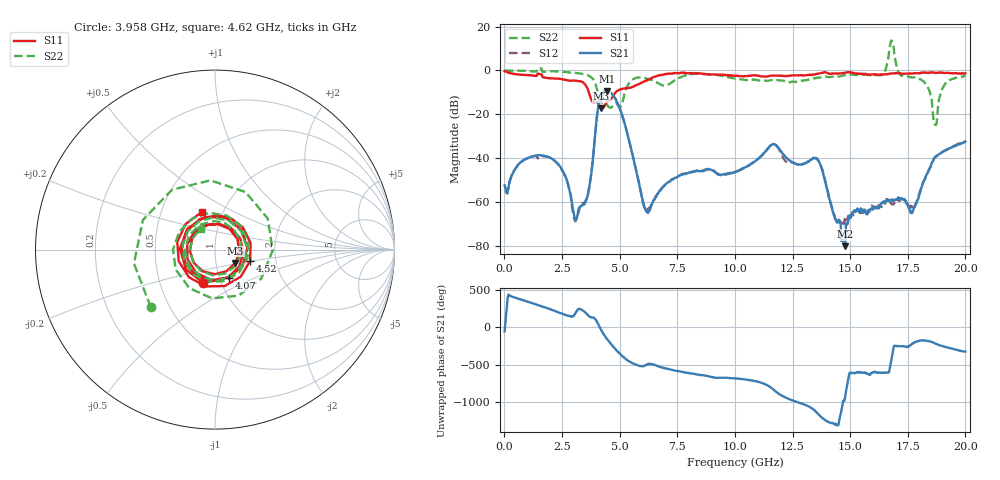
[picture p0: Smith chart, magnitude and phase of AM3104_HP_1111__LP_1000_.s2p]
!Created with skrf (http://scikit-rf.org).
# Hz S RI R 50.0
!freq ReS11 ImS11 ReS21 ImS21 ReS12 ImS12 ReS22 ImS22
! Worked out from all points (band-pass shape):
!   1601 points, 10 MHz to 20 GHz, reference 50 ohm
!   highest |S21| = -9.39 dB at 4.458 GHz (marker M1); lowest = -80.2 dB at 14.77 GHz (marker M2)
!   |S21| within 3 dB of the highest: 4.161 GHz to 4.787 GHz (625.8 MHz wide, 14 % of centre)
!   lowest |S11| = -17.3 dB at 4.208 GHz (marker M3), VSWR 1.31, Z = 62.1 - j9.4 ohm
!   |S11| at or under -10 dB: 3.665 GHz to 4.826 GHz (1.162 GHz wide, 27.4 % of centre)
!   |S22| runs from -24.9 to 13.7 dB; largest |S21 - S12| = 0.027
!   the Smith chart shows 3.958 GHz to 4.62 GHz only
!   S11 on the Smith chart (normalised r, x): 3.958 GHz: 0.82, -0.32; 4.07 GHz: 1.11, -0.36; 4.52 GHz: 1.47, -0.19; 4.62 GHz: 0.79, +0.35
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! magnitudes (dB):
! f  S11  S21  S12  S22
! 10 MHz  -0.4  -52.5  -55.0  -0.1
! 1.784 GHz  -3.3  -39.2  -39.2  -0.5
! 3.046 GHz  -4.7  -67.1  -68.3  -1.1
! 3.346 GHz  -5.1  -61.9  -60.8  -1.5
! 3.671 GHz  -10.2  -53.9  -53.8  -2.5
! 3.958 GHz  -14.2  -27.0  -26.9  -6.4
! 4.07 GHz  -15.2  -16.7  -16.8  -10.8
! 4.208 GHz  -17.3  -11.2  -11.2  -14.5
! 4.458 GHz  -14.4  -9.4  -9.4  -15.8
! 4.52 GHz  -13.8  -9.5  -9.7  -16.6
! 4.62 GHz  -13.1  -10.2  -10.3  -17.0
! 6.119 GHz  -4.8  -63.4  -63.4  -3.6
! 6.682 GHz  -2.3  -55.9  -55.9  -5.9
! 10.01 GHz  -2.5  -46.5  -46.4  -3.8
! 11.64 GHz  -2.4  -33.8  -33.7  -4.3
! 13.34 GHz  -2.1  -40.6  -40.5  -3.9
! 14.77 GHz  -1.1  -80.2  -67.8  -2.2
! 16.68 GHz  -1.6  -59.6  -59.1  7.3
! 17.71 GHz  -1.4  -64.4  -62.6  -3.2
! 18.69 GHz  -1.1  -39.4  -39.7  -24.8
! 19.1 GHz  -1.2  -36.6  -36.7  -6.4
! 20 GHz  -1.3  -32.6  -32.4  -2.6
